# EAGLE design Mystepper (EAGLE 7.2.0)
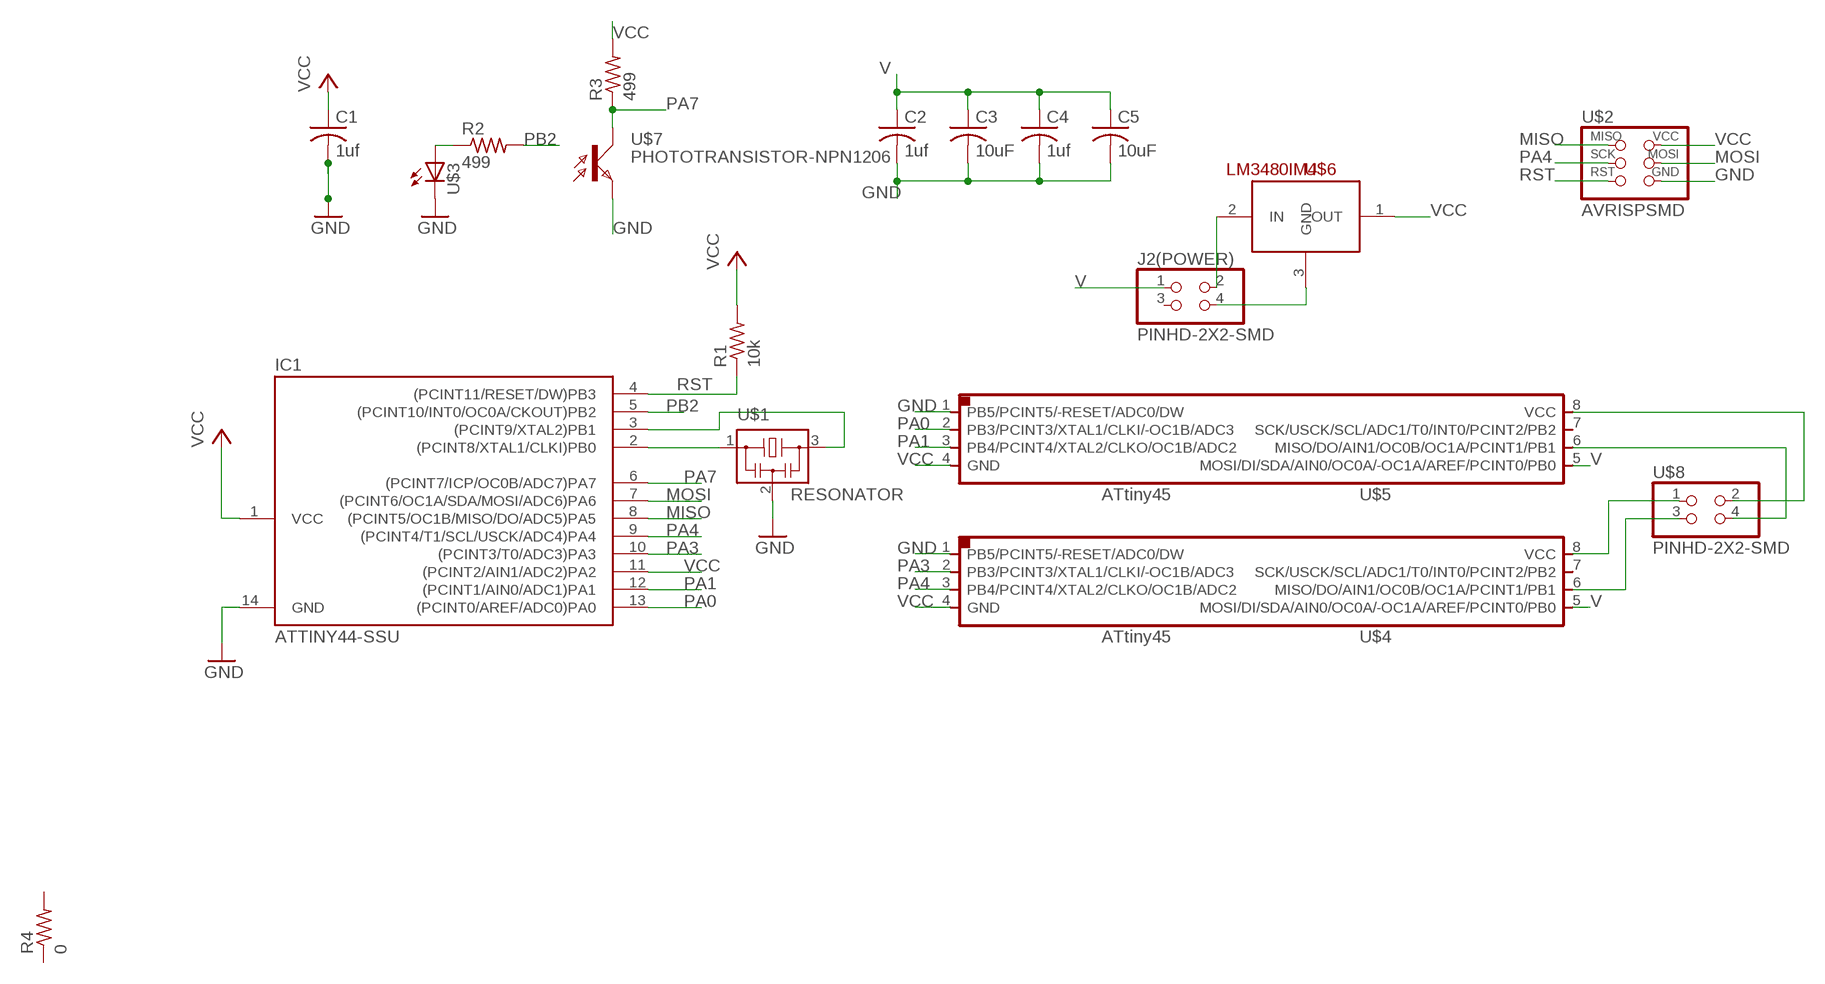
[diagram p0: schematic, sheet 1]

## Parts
C1  1uf  C-USC1206  [C1206]
C2  1uf  C-USC1206  [C1206]
C3  10uF  C-USC1206  [C1206]
C4  1uf  C-USC1206  [C1206]
C5  10uF  C-USC1206  [C1206]
IC1  ATTINY44-SSU  [SOIC14]
J2(POWER)  PINHD-2X2-SMD  [2X02SMD]
R1  10k  R-US_R1206  [R1206]
R2  499  RESISTOR1206  [1206]
R3  499  RESISTOR1206  [1206]
R4  0  RESISTOR1206  [1206]
U$1  RESONATOR  [EFOBM]
U$2  AVRISPSMD  [2X03SMD]
U$3  LED1206  [1206]
U$4  ATTINY45SI  [SOIC8]
U$5  ATTINY45SI  [SOIC8]
U$6  LM3480IM4  [SOT23-3]
U$7  PHOTOTRANSISTOR-NPN1206  [OP1206]
U$8  PINHD-2X2-SMD  [2X02SMD]

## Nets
GND: C1.2 C2.2 C3.2 C4.2 C5.2 IC1.14(GND) U$1.2 U$2.6(GND) U$3.2(C) U$4.1(PB5/PCINT5/-RESET/ADC0/DW) U$5.1(PB5/PCINT5/-RESET/ADC0/DW) U$7.EMITTER(E)
MISO: IC1.8((PCINT5/OC1B/MISO/DO/ADC5)PA5) U$2.1(MISO)
MOSI: IC1.7((PCINT6/OC1A/SDA/MOSI/ADC6)PA6) U$2.4(MOSI)
N$1: IC1.2((PCINT8/XTAL1/CLKI)PB0) U$1.1
N$2: IC1.3((PCINT9/XTAL2)PB1) U$1.3
N$3: J2(POWER).2 U$6.2(IN)
N$4: R2.1 U$3.1(A)
N$5: J2(POWER).4 U$6.3(GND)
N$6: U$5.8(VCC) U$8.2
N$7: U$5.6(MISO/DO/AIN1/OC0B/OC1A/PCINT1/PB1) U$8.4
N$8: U$4.8(VCC) U$8.1
N$9: U$4.6(MISO/DO/AIN1/OC0B/OC1A/PCINT1/PB1) U$8.3
PA0: IC1.13((PCINT0/AREF/ADC0)PA0) U$5.2(PB3/PCINT3/XTAL1/CLKI/-OC1B/ADC3)
PA1: IC1.12((PCINT1/AIN0/ADC1)PA1) U$5.3(PB4/PCINT4/XTAL2/CLKO/OC1B/ADC2)
PA3: IC1.10((PCINT3/T0/ADC3)PA3) U$4.2(PB3/PCINT3/XTAL1/CLKI/-OC1B/ADC3)
PA4: IC1.9((PCINT4/T1/SCL/USCK/ADC4)PA4) U$2.3(SCK) U$4.3(PB4/PCINT4/XTAL2/CLKO/OC1B/ADC2)
PA7: IC1.6((PCINT7/ICP/OC0B/ADC7)PA7) R3.1 U$7.COLLECTOR(C)
PB2: IC1.5((PCINT10/INT0/OC0A/CKOUT)PB2) R2.2
RST: IC1.4((PCINT11/RESET/DW)PB3) R1.1 U$2.5(RST)
V: C2.1 C3.1 C4.1 C5.1 J2(POWER).1 U$4.5(MOSI/DI/SDA/AIN0/OC0A/-OC1A/AREF/PCINT0/PB0) U$5.5(MOSI/DI/SDA/AIN0/OC0A/-OC1A/AREF/PCINT0/PB0)
VCC: C1.1 IC1.1(VCC) IC1.11((PCINT2/AIN1/ADC2)PA2) R1.2 R3.2 U$2.2(VCC) U$4.4(GND) U$5.4(GND) U$6.1(OUT)
Unconnected: J2(POWER).3 R4.1 R4.2 U$4.7(SCK/USCK/SCL/ADC1/T0/INT0/PCINT2/PB2) U$5.7(SCK/USCK/SCL/ADC1/T0/INT0/PCINT2/PB2)

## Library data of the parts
C1-C5 = rcl:C-US: CAPACITOR, American symbol
IC1 = fab:ATTINY44
J2(POWER) U$8 = fab:PINHD-2X2-SMD
R1 = resistor:R-US_: RESISTOR, American symbol
R2-R4 = 01_FAB_Hello:RESISTOR
U$1 = fab:RESONATOR
U$2 = fab:AVRISP
U$3 = 01_FAB_Hello:LED
U$4 U$5 = fab:ATTINY45
U$6 = SparkFun-PowerIC:LM3480IM4: Small package linear regulator
U$7 = fab:PHOTOTRANSISTOR-NPN

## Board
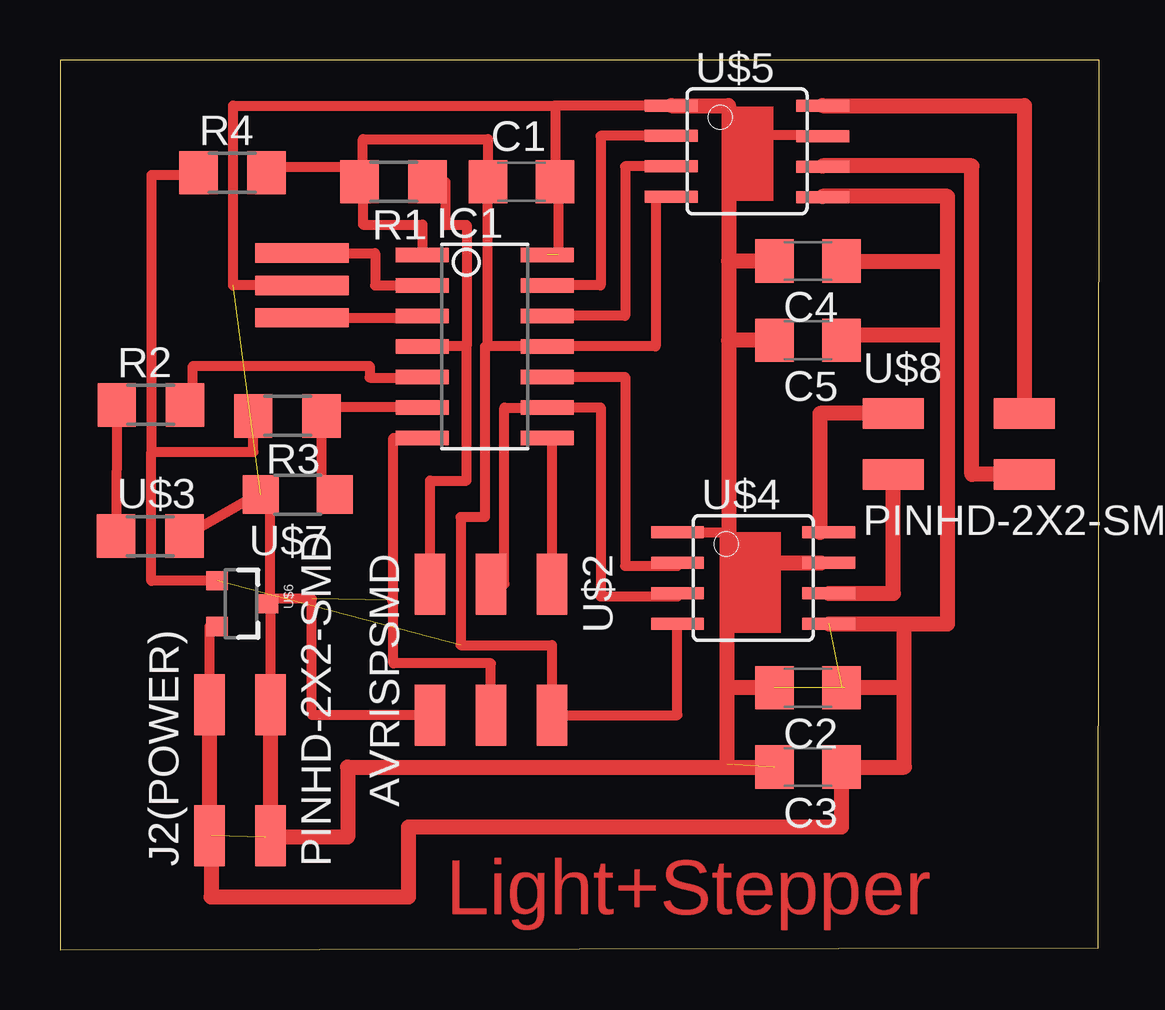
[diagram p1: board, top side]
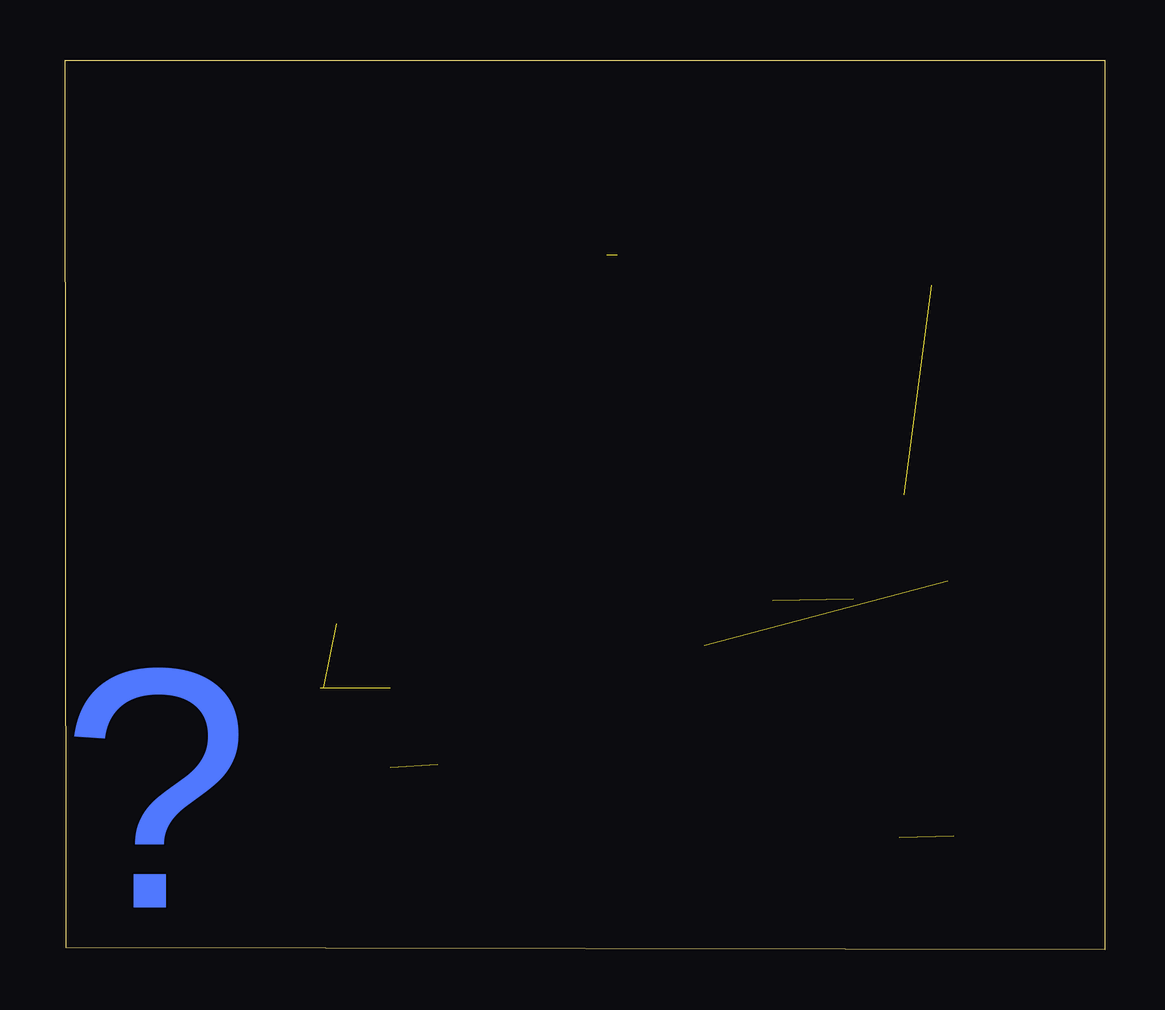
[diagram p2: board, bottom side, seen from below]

Size 43.31 x 37.07 mm. Coordinates in mm from the lower left corner, seen from the top.
Outline: 0,0 43.27,0.08 43.31,37.06 0.01,37.07 0,0
Copper layers 1: Top 0.035mm
Design rules "ERP-1sided-10mil-16mill": minimum track width 10mil, minimum drill 24mil, track to track 16mil, track to pad 16mil, pad to pad 16mil, via to via 16mil, smd to smd 0mil, copper to edge 16mil, drill to drill 36mil, minimum pad ring 10mil, minimum via ring 8mil, stop-mask expansion 4mil, vias tented up to drill 0mil, thermal gap 10mil

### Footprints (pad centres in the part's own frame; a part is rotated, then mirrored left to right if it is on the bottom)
C1206 = smd 1.6 x 1.8: 1 -1.4,0; 2 1.4,0
SOIC14 = smd 0.61 x 2.21: 1 -3.81,-2.603; 2 -2.54,-2.603; 3 -1.27,-2.603; 4 0,-2.603; 5 1.27,-2.603; 6 2.54,-2.603; 7 3.81,-2.603; 8 3.81,2.603; 9 2.54,2.603; 10 1.27,2.603; 11 0,2.603; 12 -1.27,2.603; 13 -2.54,2.603; 14 -3.81,2.603
2X02SMD = smd 2.54 x 1.27: 1 -2.54,1.27; 2 2.92,1.27; 3 -2.54,-1.27; 4 2.92,-1.27
R1206 = smd 1.6 x 1.803: 1 -1.422,0; 2 1.422,0
1206 = smd 1.6 x 1.803: 1 -1.422,0; 2 1.422,0
EFOBM = smd 0.8 x 3.9: 1 -1.35,0; 2 0,0; 3 1.35,0
2X03SMD = smd 2.54 x 1.27: 1 -2.54,2.54; 2 2.92,2.54; 3 -2.54,0; 4 2.92,0; 5 -2.54,-2.54; 6 2.92,-2.54
SOIC8 = smd 0.5 x 2.2: 1 -1.905,-3.154; 2 -0.645,-3.154; 3 0.625,-3.154; 4 1.895,-3.154; 5 1.905,3.154; 6 0.635,3.154; 7 -0.635,3.154; 8 -1.905,3.154
SOT23-3 = smd 0.8 x 0.9: 1 -0.95,-1; 2 0.95,-1; 3 0,1.1
OP1206 = smd 1.5 x 1.6: COLLECTOR -1.55,0; EMITTER 1.55,0

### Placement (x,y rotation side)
C1  19.23,31.99 0 top
C2  31.17,10.91 180 top
C3  31.17,7.61 180 top
C4  31.17,28.69 180 top
C5  31.17,25.39 180 top
IC1  17.7,25.13 270 top
J2(POWER)  7.49,7.28 90 top
R1  13.89,31.99 180 top
R2  3.78,22.69 0 top
R3  9.47,22.24 180 top
R4  7.19,32.37 0 top
U$1  10.08,27.67 270 top
U$2  17.96,12.69 270 top
U$3  3.76,17.23 0 top
U$4  28.88,15.48 270 top
U$5  28.63,33.26 270 top
U$6  7.54,14.41 270 top
U$7  9.91,18.96 180 top
U$8  37.26,21.07 0 top

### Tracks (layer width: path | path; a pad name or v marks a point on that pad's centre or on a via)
GND  (5 unrouted)
  Top 0.406: U$5.1 20.63,35.17 | 20.63,35.17 C1.2 20.75,31.99 20.75,28.94 | U$4.1 27.79,17.39 27.86,17.39 | 35.08,10.91 35.08,11.09 | 32.69,10.91 32.69,11.04 | 8.74,14.62 8.74,18.94 U$7.EMITTER 7.9,18.78 U$3.2 | 13.84,14.57 13.84,14.67 | U$2.6 10.49,9.77 10.49,14.62 8.74,14.62 | 8.74,14.62 8.74,14.57 | U$1.2 7.21,27.67 7.21,35.17 20.63,35.17
  Top 0.635: U$5.1 27.86,35.17 27.86,28.69 | 27.86,28.69 27.86,25.39 | C4.2 27.86,28.69 | C5.2 27.86,25.39 | 27.86,25.39 27.86,17.39 | 27.79,17.39 27.79,10.91 | 27.79,10.91 27.79,7.73 | C2.2 27.79,10.91 | 35.08,10.91 32.69,10.91
MISO
  Top 0.406: IC1.8 20.5,21.32 U$2.1
MOSI
  Top 0.406: 14.91,21.32 IC1.7 13.89,21.32 13.89,11.93 17.96,11.93 U$2.4
N$1
  Top 0.406: U$1.1 13.13,29.02 13.13,27.67 IC1.2
N$2
  Top 0.406: U$1.3 15.1,26.32 IC1.3
N$3
  Top 0.406: U$6.2 6.22,13.46 J2(POWER).2
N$4
  Top 0.406: 2.36,23.15 R2.1 U$3.1
N$5
  Top 0.406: U$6.3 8.76,14.41 J2(POWER).4
N$6
  Top 0.635: U$5.8 40.18,35.17 U$8.2
N$7
  Top 0.406: 31.78,32.65 U$5.6
  Top 0.635: U$8.4 38,19.8 38,32.65 31.78,32.65
N$8
  Top 0.406: U$4.8 31.67,17.39
  Top 0.635: 31.67,17.39 31.67,22.34 U$8.1
N$9
  Top 0.635: U$4.6 34.72,14.85 U$8.3
N$10
  Top 0.406: 31.7,16.12 31.7,16.19
  Top 0.635: 27.86,16.12 31.7,16.12
N$11
  Top 0.406: 27.97,33.95 31.67,33.95
N$12
  Top 0.406: 8.99,32.63 12.65,32.63 12.65,32.5
PA0
  Top 0.406: U$5.2 22.53,33.91 22.53,27.67 IC1.13
PA1
  Top 0.406: U$5.3 23.55,32.64 23.55,26.4 IC1.12
PA3
  Top 0.406: IC1.10 23.55,23.86 23.55,15.99 25.73,15.99 U$4.2
PA4
  Top 0.406: U$4.3 25.73,14.72 22.53,14.72 22.53,22.59 IC1.9 20.31,22.58 18.52,22.58 18.52,15.23 U$2.3
PA7
  Top 0.406: IC1.6 10.9,22.59 R3.1 10.9,19.04 11.02,19.04 11.02,18.94 U$7.COLLECTOR
PB2
  Top 0.406: R2.2 5.54,22.16 5.54,24.32 12.9,24.32 12.9,23.84 15.1,23.84 IC1.5
RST
  Top 0.406: U$2.5 15.42,19.55 16.94,19.55 16.94,25.13 | 16.94,25.13 IC1.4 | R1.1 16.06,31.99 16.06,30.2 16.94,30.2 16.94,25.13
V  (2 unrouted)
  Top 0.406: 31.78,31.38 U$5.5 | C5.1 32.69,25.39 32.69,25.62 | J2(POWER).1 6.25,4.74 6.3,4.74 | 29.87,7.61 29.87,7.58 | 8.56,4.69 8.79,4.69
  Top 0.635: U$4.5 35.18,13.58 | 35.18,13.58 36.98,13.58 36.98,25.62 | 36.98,25.62 36.98,28.69 | 36.98,28.69 36.98,31.38 31.78,31.38 | C4.1 36.98,28.69 | 32.69,25.62 36.98,25.62 | 6.3,4.74 6.3,2.2 14.53,2.2 14.53,5.12 32.57,5.12 C3.1 35.18,7.61 35.18,13.58 | 29.87,7.61 11.99,7.61 11.99,4.69 8.79,4.69 8.79,10.2 | 6.25,4.74 6.25,10.2
VCC  (1 unrouted)
  Top 0.406: R1.2 12.62,31.99 | 12.62,31.99 12.62,30.21 15.1,30.21 IC1.1 | 12.62,31.99 12.62,33.77 17.83,33.77 C1.1 17.83,25.13 | U$5.4 24.82,31.37 24.82,25.13 IC1.11 17.83,25.13 | U$4.4 25.73,9.77 U$2.2 20.5,12.69 16.69,12.69 16.69,18.02 17.7,18.02 17.7,25.13 17.83,25.13 | U$6.1 3.81,15.36 3.81,20.61 3.81,20.74 | 3.81,20.74 8.05,20.74 R3.2 | 5.71,32.27 3.81,32.27 3.81,20.74
(copper drawn outside any net)
  shapes: Top area x2

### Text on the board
Top: Light+Stepper
Bottom: ?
